(* Logix 5000 AddOnInstructionDefinition export wxsHeartbeat_v01; software revision 30.02 *)

ADD_ON_INSTRUCTION wxsHeartbeat_v01   (* revision 1.0, vendor Pendant Automation *)
// Heartbeat AOI for WXS Middleware
VAR_INPUT
   TimeoutSetpoint : INT; {required}   // Timeout Setpoint (miliseconds)
   TxHeartbeat : BOOL; {required}
   RxHeartbeat : BOOL; {required}
   DivertConfirmHeartbeat : BOOL; {required}
END_VAR
VAR_OUTPUT
   TxLossOfComms : BOOL; {access Read Only, visible}
   RxLossOfComms : BOOL; {access Read Only, visible}
   DivertConfirmLossOfComms : BOOL; {access Read Only, visible}
END_VAR
VAR_INPUT
   DisableDivertConfirm : BOOL; {required}   // 0 to Enable 1 to Disable
END_VAR
VAR
   tmrTxHeartbeat_True : TIMER; {access None}
   tmrTxHeartbeat_False : TIMER; {access None}
   tmrRxHeartbeat_True : TIMER; {access None}
   tmrRxHeartbeat_False : TIMER; {access None}
   tmrDivertConfirmHeartbeat_True : TIMER; {access None}
   tmrDivertConfirmHeartbeat_False : TIMER; {access None}
END_VAR

ROUTINE Logic   (* ladder *)
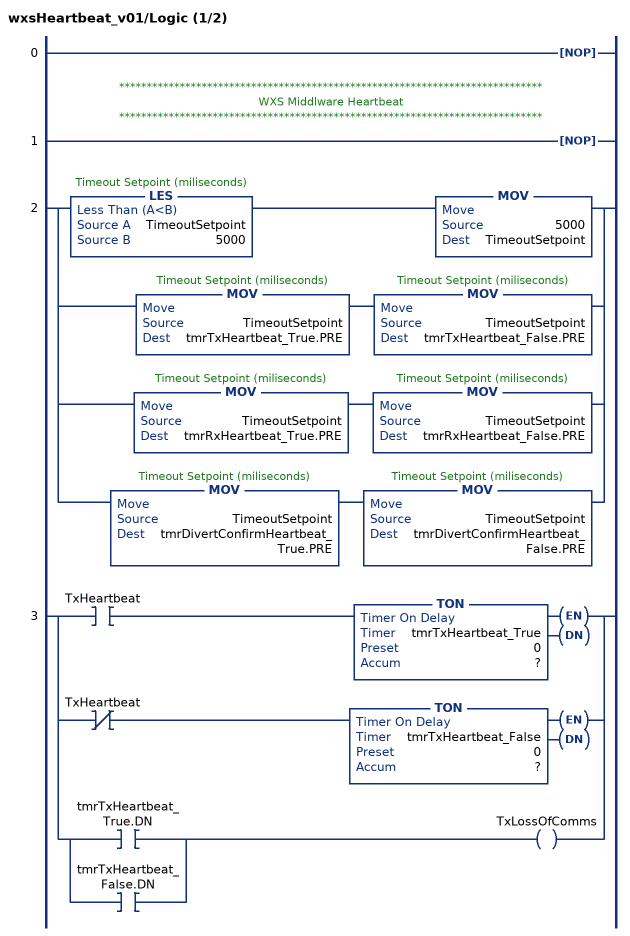
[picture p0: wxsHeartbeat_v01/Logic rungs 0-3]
   0: NOP();
   // *****************************************************************************
   // WXS Middlware Heartbeat
   // *****************************************************************************
   1: NOP();
   2: [LES(TimeoutSetpoint,5000) MOV(5000,TimeoutSetpoint) ,MOV(TimeoutSetpoint,tmrTxHeartbeat_True.PRE) MOV(TimeoutSetpoint,tmrTxHeartbeat_False.PRE) ,MOV(TimeoutSetpoint,tmrRxHeartbeat_True.PRE) MOV(TimeoutSetpoint,tmrRxHeartbeat_False.PRE) ,MOV(TimeoutSetpoint,tmrDivertConfirmHeartbeat_True.PRE) MOV(TimeoutSetpoint,tmrDivertConfirmHeartbeat_False.PRE) ];
   3: [XIC(TxHeartbeat) TON(tmrTxHeartbeat_True,?,?) ,XIO(TxHeartbeat) TON(tmrTxHeartbeat_False,?,?) ,[XIC(tmrTxHeartbeat_True.DN) ,XIC(tmrTxHeartbeat_False.DN) ] OTE(TxLossOfComms) ];
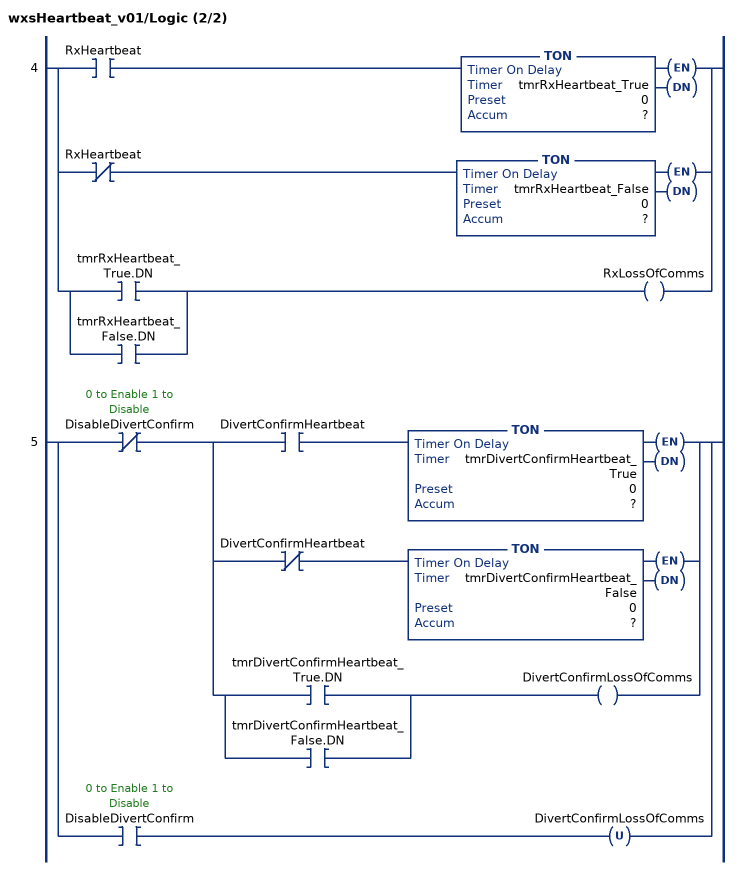
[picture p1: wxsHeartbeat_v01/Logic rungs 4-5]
   4: [XIC(RxHeartbeat) TON(tmrRxHeartbeat_True,?,?) ,XIO(RxHeartbeat) TON(tmrRxHeartbeat_False,?,?) ,[XIC(tmrRxHeartbeat_True.DN) ,XIC(tmrRxHeartbeat_False.DN) ] OTE(RxLossOfComms) ];
   5: [XIO(DisableDivertConfirm) [XIC(DivertConfirmHeartbeat) TON(tmrDivertConfirmHeartbeat_True,?,?) ,XIO(DivertConfirmHeartbeat) TON(tmrDivertConfirmHeartbeat_False,?,?) ,[XIC(tmrDivertConfirmHeartbeat_True.DN) ,XIC(tmrDivertConfirmHeartbeat_False.DN) ] OTE(DivertConfirmLossOfComms) ] ,XIC(DisableDivertConfirm) OTU(DivertConfirmLossOfComms) ];
END_ROUTINE
END_ADD_ON_INSTRUCTION
